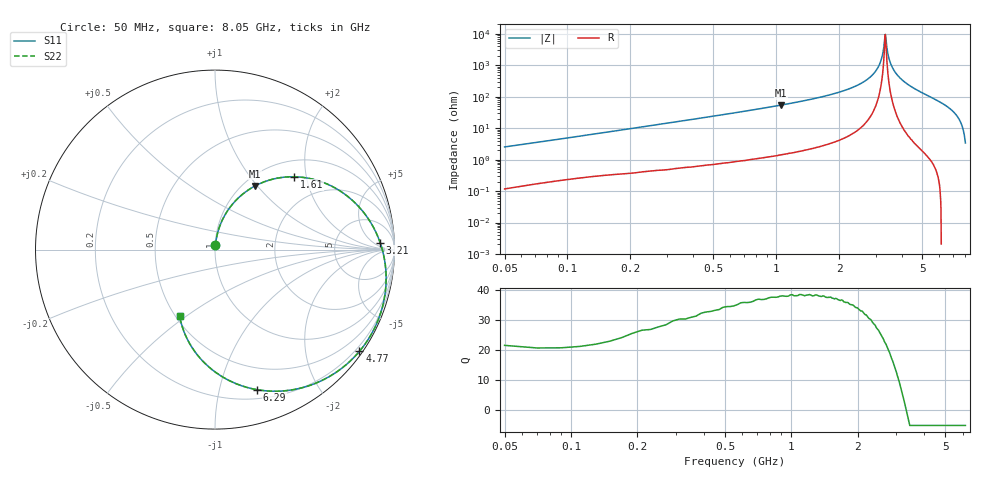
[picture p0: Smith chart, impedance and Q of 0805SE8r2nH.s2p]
! AVX Thin Film Operation		Date: May 2002
! Description: Accu-L® Series, Thin Film, SMD, RF Inductors
! Part Number: L08058R2CEWTR
! 50 MHz  -  8.05 GHz
! Serial Measurements
# mhz S db R 50
!	S11		S21		S12		S22
!	dB	Phase	dB	Phase	dB	Phase	dB	Phase
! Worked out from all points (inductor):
!   401 points, 50 MHz to 8.05 GHz, reference 50 ohm
!   read as 1/Y11, port 2 shorted: L = 7.72 nH near 90 MHz
!   highest Q = 38.3 at 1.05 GHz (marker M1), where L = 8.18 nH
!   self-resonance near 3.31 GHz
!   S11 on the Smith chart (normalised r, x): 50 MHz: 1.00, +0.05; 1.61 GHz: 1.34, +1.70; 3.21 GHz: 19, +10; 4.77 GHz: 0.09, -3.16; 6.29 GHz: 0.28, -1.30; 8.05 GHz: 0.53, -0.47
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50  -32.76 85.1  -0.01 -1.6  -0.01 -1.6  -32.76 85.1
170  -22.63 82.3  -0.05 -5.1  -0.05 -5.1  -22.63 82.3
350  -16.55 77.5  -0.14 -10.4  -0.14 -10.4  -16.55 77.5
630  -11.65 69.7  -0.37 -18.4  -0.37 -18.4  -11.65 69.7
1050  -7.57 57.9  -0.93 -30.2  -0.93 -30.2  -7.57 57.9
1390  -5.48 48.6  -1.56 -39.4  -1.56 -39.4  -5.48 48.6
1610  -4.45 42.6  -2.06 -45.2  -2.06 -45.2  -4.45 42.6
2730  -1.38 14.1  -5.99 -72.8  -5.99 -72.8  -1.38 14.1
3210  -0.71 2.4  -8.78 -83.9  -8.78 -83.9  -0.71 2.4
3710  -0.29 -9.6  -13.35 -94.6  -13.35 -94.6  -0.29 -9.6
4050  -0.14 -17.7  -19.07 -100.2  -19.07 -100.2  -0.14 -17.7
4230  -0.10 -22.0  -25.00 -99.2  -25.00 -99.2  -0.10 -22.0
4310  -0.09 -24.0  -29.80 -90.4  -29.80 -90.4  -0.09 -24.0
4370  -0.08 -25.4  -35.40 -56.8  -35.40 -56.8  -0.08 -25.4
4410  -0.08 -26.4  -38.90 -31.3  -38.90 -31.3  -0.08 -26.4
4590  -0.09 -30.8  -24.86 53.1  -24.86 53.1  -0.09 -30.8
4770  -0.14 -35.1  -18.94 53.6  -18.94 53.6  -0.14 -35.1
5030  -0.25 -41.5  -14.26 49.3  -14.26 49.3  -0.25 -41.5
5390  -0.51 -50.5  -10.34 41.7  -10.34 41.7  -0.51 -50.5
6290  -1.78 -73.3  -5.01 20.5  -5.01 20.5  -1.78 -73.3
6730  -2.77 -84.6  -3.48 10.0  -3.48 10.0  -2.77 -84.6
8050  -7.56 -118.1  -0.97 -20.3  -0.97 -20.3  -7.56 -118.1
